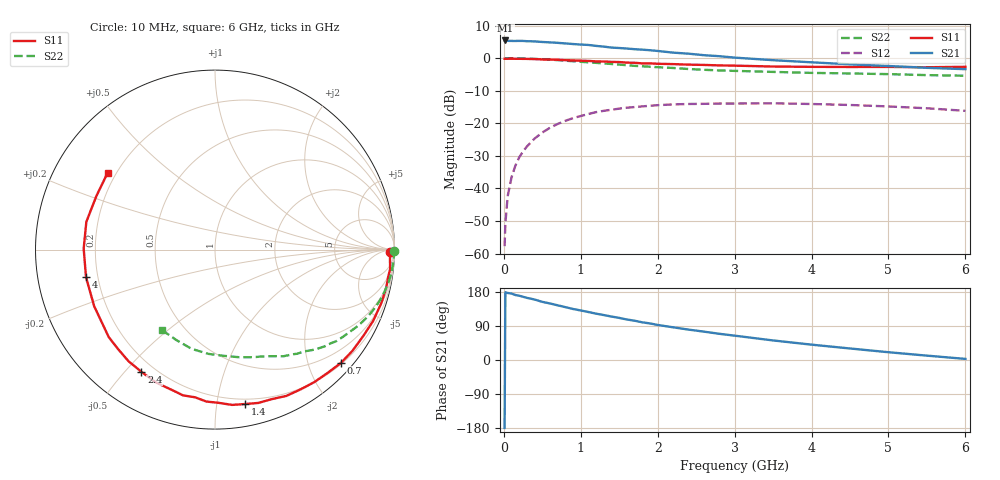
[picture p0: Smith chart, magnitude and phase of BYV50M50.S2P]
! SIEMENS Small Signal Semiconductors
! BFY420
! Si NPN RF SIEGET Grounded Emitter Transistor in MICRO-X
! VCE = 0.5 V  IC = 0.5 mA
! Common Emitter S-Parameters:  October  1996
# GHz  S  MA  R  50
!  f  S11  S21  S12  S22
! GHz  MAG  ANG  MAG  ANG  MAG  ANG  MAG  ANG
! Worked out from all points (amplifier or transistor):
!   36 points, 10 MHz to 6 GHz, reference 50 ohm
!   highest |S21| = 5.4 dB at 20 MHz (marker M1)
!   |S21| within 3 dB of that: start of sweep to 1.898 GHz
!   unconditionally stable (mu >= 1): 4.666 GHz to end of sweep
!   at 250 MHz: K = 0.05, MSG = 17.0 dB, |S12| = -28.6 dB
!   at 1.4 GHz: K = 0.25, MSG = 9.5 dB, |S12| = -15.8 dB
!   at 6 GHz: K = 1.36, MAG = 2.8 dB, |S12| = -16.2 dB
!   S11 on the Smith chart (normalised r, x): 10 MHz: 68, -36; 700 MHz: 0.22, -2.60; 1.4 GHz: 0.16, -1.20; 2.4 GHz: 0.15, -0.55; 4 GHz: 0.15, -0.10; 6 GHz: 0.17, +0.31
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0.01  0.9773 -0.7  1.853 -179.3  0.0013 97.0  0.9995 -0.4
0.02  0.9762 -1.2  1.868 178.8  0.0029 92.1  0.9916 -0.7
0.05  0.9763 -3.1  1.842 176.9  0.0076 87.4  0.9986 -1.7
0.1  0.9818 -6.3  1.837 175.2  0.0148 86.1  0.9954 -3.5
0.15  0.9766 -9.0  1.834 171.5  0.0224 82.9  0.9939 -5.3
0.2  0.9773 -12.2  1.84 169.6  0.03 82.3  0.9924 -7.0
0.3  0.9734 -17.9  1.82 164.0  0.0441 77.9  0.9848 -10.4
0.4  0.9665 -24.3  1.807 159.6  0.0583 73.6  0.9737 -13.8
0.5  0.956 -30.4  1.77 153.4  0.0721 69.6  0.9623 -17.0
0.7  0.9441 -41.9  1.717 144.3  0.0977 61.8  0.9315 -23.3
0.9  0.9227 -53.1  1.647 134.6  0.12 54.0  0.8961 -29.0
1.1  0.9069 -64.0  1.594 126.6  0.139 46.9  0.8621 -34.4
1.4  0.8764 -79.0  1.452 114.7  0.1616 37.1  0.8136 -41.6
1.8  0.8303 -97.7  1.35 99.4  0.1817 26.2  0.7504 -49.5
2.2  0.8102 -113.9  1.215 86.3  0.195 16.1  0.7067 -57.2
2.4  0.7947 -121.1  1.171 80.2  0.1978 12.2  0.681 -60.7
2.8  0.7735 -134.4  1.071 69.2  0.2011 4.5  0.6474 -67.0
3.5  0.7434 -154.9  0.93 51.6  0.2026 -6.5  0.6147 -77.3
4  0.7349 -167.9  0.863 40.5  0.1977 -13.5  0.5937 -85.4
4.5  0.7317 179.6  0.803 30.4  0.191 -19.8  0.5821 -93.6
5.5  0.7252 155.7  0.71 11.5  0.17 -30.2  0.5487 -112.8
6  0.7354 144.4  0.677 2.9  0.1553 -33.4  0.5367 -123.4
